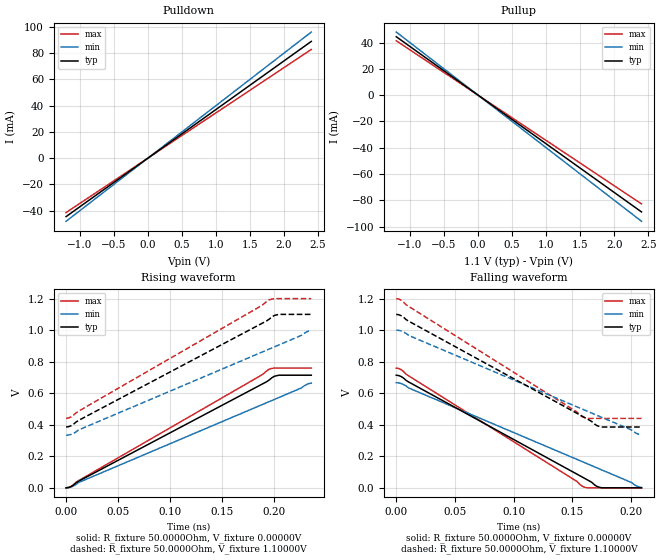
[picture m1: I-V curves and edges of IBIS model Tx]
[IBIS Ver]   5.1
[File name]   spisimami.ibs
[File rev]   1.00
[Date]   Jan 1, 2017
[Source]   BPro (http://www.spisim.com)
[Copyright]   Copyright 2017 ~, SPISim LLC. All right reserved.
[Component]   Spec_Model
[Manufacturer]  SPISim LLC
[Package]
|   typ   min   max
R_pkg   0.0   0.0   0.0
L_pkg   0.0   0.0   0.0
C_pkg   0.0   0.0   0.0
[PIN]   signal_name   model_name   R_pin   L_pin   C_pin
1p   TxP   Tx   NA   NA   NA
1n   TxN   Tx   NA   NA   NA
2p   RxP   Rx   NA   NA   NA
2n   RxN   Rx   NA   NA   NA
[Diff Pin] inv_pin  vdiff  tdelay_typ  tdelay_min  tdelay_max
1p   1n   0.1V   NA   NA   NA
2p   2n   0.1V   NA   NA   NA
[Model]   Rx
Model_type  Input
C_comp 0.00p 0.00p 0.00p
Vinh = 0.55
Vinl = 0.45
[Temperature_Range]  25   100   0
[Voltage Range]   1.2   1.14  1.26
[Algorithmic Model]
Executable Windows_VisualStudio_32 SPISimAMI_WIN32.dll IBIS_AMI_TX.ami
Executable Windows_VisualStudio_64 SPISimAMI_WIN64.dll IBIS_AMI_TX.ami
Executable Linux_gcc_64   SPISimAMI_LX64.so   IBIS_AMI_TX.ami
[End Algorithmic Model]
| Models and submodels in the file (2): Rx (Input), Tx (Output)
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[Model]   Tx
Model_type   Output
Polarity   Non-Inverting
Enable   Active-High
Vmeas =   0.55
|   typ   min   max
C_comp   2.0pF   1.5pF   2.5pF
[Voltage Range]   1.1   1.0   1.2
[Temperature Range]   60   100   0
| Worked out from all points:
|   slope of the pulldown table from 0 to 0.165 V, typ, clamps not added: 27 ohm
|   slope of the pullup table from 0 to 0.165 V, typ, clamps not added: 27 ohm
|   rising waveform, R_fixture 50.0000Ohm, V_fixture 0.00000V: 20-80 % time 123ps typ, 143ps min, 120ps max; typ from 0 V to 0.714 V
|   falling waveform, R_fixture 50.0000Ohm, V_fixture 0.00000V: 20-80 % time 105ps typ, 126ps min, 97.6ps max; typ from 0.714 V to 0 V
|   rising waveform, R_fixture 50.0000Ohm, V_fixture 1.10000V: 20-80 % time 123ps typ, 143ps min, 120ps max; typ from 0.386 V to 1.1 V
|   falling waveform, R_fixture 50.0000Ohm, V_fixture 1.10000V: 20-80 % time 105ps typ, 126ps min, 97.6ps max; typ from 1.1 V to 0.386 V
[Pullup]
| Voltage I(typ) I(min) I(max)
-1.2V     44.44mA    48mA       41.38mA
0V        0A         0A         0A
2.4V      -88.89mA   -96mA      -82.76mA
[Pulldown]
| Voltage I(typ) I(min) I(max)
-1.2V     -44.44mA   -48mA      -41.38mA
0V        0A         0A         0A
2.4V      88.89mA    96mA       82.76mA
[Rising Waveform]
R_fixture = 50.0000Ohm
V_fixture = 0.00000V
V_fixture_min = 0.00000V
V_fixture_max = 0.00000V
|   TIME   V(TYP)   V(MIN)   V(MAX)
0s        0V         0V         0V
4.772ps   8.052mV    5.333mV    9.008mV
11.93ps   41.56mV    33.33mV    45.31mV
188.5ps   656.6mV    526.7mV    715.8mV
195.7ps   683.9mV    546.7mV    752.1mV
200.4ps   706.7mV    560mV      759.5mV
205.2ps   714.3mV    573.3mV    759.5mV
226.7ps   714.3mV    633.3mV    759.5mV
231.5ps   714.3mV    654.7mV    759.5mV
236.2ps   714.3mV    664mV      759.5mV
[Falling Waveform]
R_fixture = 50.0000Ohm
V_fixture = 0.00000V
V_fixture_min = 0.00000V
V_fixture_max = 0.00000V
|   TIME   V(TYP)   V(MIN)   V(MAX)
0s        714.3mV    666.7mV    759.5mV
4.222ps   705.6mV    661.3mV    748.9mV
8.444ps   680.9mV    645.3mV    720.1mV
10.56ps   671.3mV    633.3mV    710.2mV
154.1ps   86.33mV    180mV      39.91mV
158.3ps   69.12mV    166.7mV    11.08mV
162.6ps   51.92mV    153.3mV    191.8uV
171ps     8.94mV     126.7mV    0V
175.2ps   122.9uV    113.3mV    0V
209ps     0V         2.667mV    0V
[Rising Waveform]
R_fixture = 50.0000Ohm
V_fixture = 1.10000V
V_fixture_min = 1.00000V
V_fixture_max = 1.20000V
|   TIME   V(TYP)   V(MIN)   V(MAX)
0s        385.7mV    333.3mV    440.5mV
4.772ps   393.8mV    338.7mV    449.5mV
11.93ps   427.3mV    366.7mV    485.8mV
188.5ps   1.042V     860mV      1.156V
195.7ps   1.07V      880mV      1.193V
200.4ps   1.093V     893.3mV    1.2V
205.2ps   1.1V       906.7mV    1.2V
226.7ps   1.1V       966.7mV    1.2V
231.5ps   1.1V       988mV      1.2V
236.2ps   1.1V       997.3mV    1.2V
[Falling Waveform]
R_fixture = 50.0000Ohm
V_fixture = 1.10000V
V_fixture_min = 1.00000V
V_fixture_max = 1.20000V
|   TIME   V(TYP)   V(MIN)   V(MAX)
0s        1.1V       1V         1.2V
4.222ps   1.091V     994.7mV    1.189V
8.444ps   1.067V     978.7mV    1.161V
10.56ps   1.057V     966.7mV    1.151V
154.1ps   472mV      513.3mV    480.4mV
158.3ps   454.8mV    500mV      451.6mV
162.6ps   437.6mV    486.7mV    440.7mV
171ps     394.7mV    460mV      440.5mV
175.2ps   385.8mV    446.7mV    440.5mV
209ps     385.7mV    336mV      440.5mV
[Ramp]
R_load = 50.0Ohm
|   typ   min   max
dV/dt_r   2.40E-1V/6.89E-2ns  2.40E-1V/8.59E-2ns  2.40E-1V/6.32E-2ns
dV/dt_f   2.40E-1V/5.89E-2ns  2.40E-1V/7.60E-2ns  2.40E-1V/5.14E-2ns
[Algorithmic Model]
Executable Windows_VisualStudio_32 SPISimAMI_WIN32.dll IBIS_AMI_TX.ami
Executable Windows_VisualStudio_64 SPISimAMI_WIN64.dll IBIS_AMI_TX.ami
Executable Linux_gcc_64   SPISimAMI_LX64.so   IBIS_AMI_TX.ami
[End Algorithmic Model]
